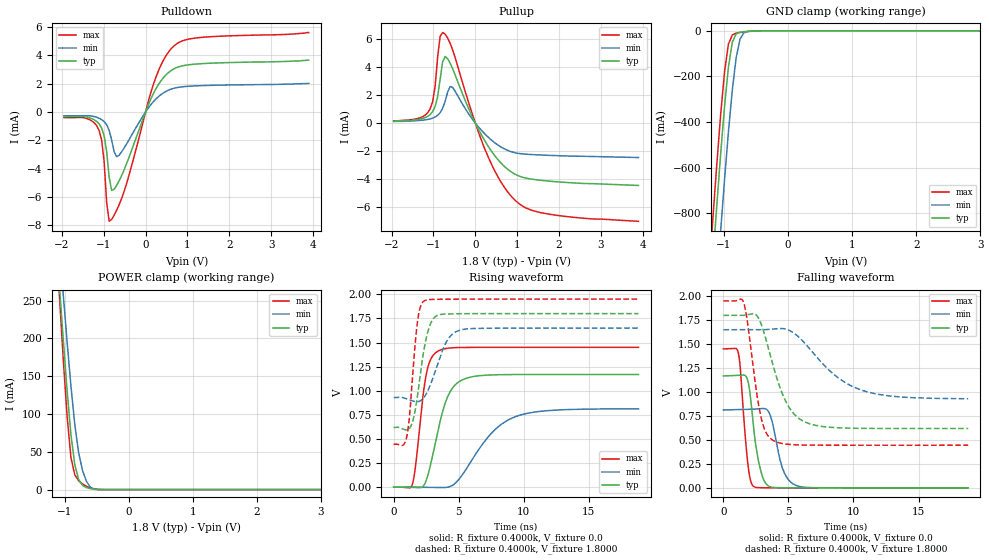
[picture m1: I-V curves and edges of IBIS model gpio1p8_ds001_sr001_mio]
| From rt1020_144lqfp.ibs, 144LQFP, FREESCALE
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[Model] gpio1p8_ds001_sr001_mio
|   Model gpio1p8_ds001_sr001_mio
| This model was characterised for following simulation conditions:
| External (pad) voltage:
|   - Typ: 1.8V,   - Min: 1.65V,   - Max: 1.95V
| Library cells for typ/min/max conditions are connected as defined below:
|  pad - External Pad
|  ipp_do - Core Input
|  ipp_obe - Output Buffer Enable
|  esd_boost - ovdd
|  ipp_dse0 - vddi
|  ipp_dse1 - vssi
|  ipp_dse2 - vssi
|  ipp_fsel0 - vddi
|  ipp_fsel1 - vssi
|  ipp_ina - ipp_ina
|  ipp_ind - ipp_ind
|  ipp_pwr_stable - vddi
|  ipp_sre - vssi
|  ovdd - ovdd
|  ovss - ovss
|  vddi - vddi
|  vssi - vssi
| All other pins connected to ground
Model_type I/O
Polarity   Non-Inverting
Enable   Active-High
Vinl =   0.5400V
Vinh =   1.2600V
Vmeas =  0.9000V
Cref =   0.0F
Rref =   0.4000k
Vref =   0.9000V
C_comp   1.2573pF   1.2208pF   1.3054pF
|C_comp_pullup   0.6439pF   0.6609pF   0.6284pF
|C_comp_pulldown   0.5473pF   0.5786pF   0.5258pF
[Model Spec]
| variable   typ   min   max
Vinh   1.2600V   1.1550V   1.3650V
Vinl   0.5400V   0.4950V   0.5850V
S_overshoot_high   1.8000V   1.6500V   1.9500V
S_overshoot_low   0.0V   0.0V   0.0V
Vmeas   0.9000V   0.8250V   0.9750V
Vref   0.9000V   0.8250V   0.9750V
Cref   0.0F   0.0F   0.0F
Rref   0.4000k   0.4000k   0.4000k
[Temperature Range]   25.0000   0.1050k   -20.0000
[Voltage Range]   1.8000V   1.6500V   1.9500V
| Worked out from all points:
|   slope of the pulldown table from 0 to 0.27 V, typ, clamps not added: 153 ohm
|   slope of the pullup table from 0 to 0.27 V, typ, clamps not added: 182 ohm
|   GND clamp passes 1 mA (typ) near -0.55 V on its own axis
|   POWER clamp passes 1 mA (typ) near -0.58 V on its own axis
|   rising waveform, R_fixture 0.4000k, V_fixture 0.0: 20-80 % time 1.3ns typ, 2.8ns min, 747ps max; typ from 0 V to 1.17 V
|   rising waveform, R_fixture 0.4000k, V_fixture 1.8000: 20-80 % time 809ps typ, 1.19ns min, 547ps max; typ from 0.619 V to 1.8 V
|   falling waveform, R_fixture 0.4000k, V_fixture 0.0: 20-80 % time 681ps typ, 847ps min, 496ps max; typ from 1.17 V to 0 V
|   falling waveform, R_fixture 0.4000k, V_fixture 1.8000: 20-80 % time 1.74ns typ, 3.41ns min, 947ps max; typ from 1.8 V to 0.619 V
[Pulldown]
|Voltage   I(typ)   I(min)   I(max)
-1.95V    -342uA     -265uA     -391uA
-1.41V    -350uA     -258uA     -451uA
-1.11V    -834.5uA   -436uA     -1.299mA
-990mV    -1.66mA    -669.8uA   -3.467mA
-930mV    -2.764mA   -895.4uA   -6.362mA
-870mV    -4.603mA   -1.287mA   -7.724mA
-810mV    -5.539mA   -1.972mA   -7.596mA
-750mV    -5.458mA   -2.817mA   -7.285mA
-630mV    -4.849mA   -3.046mA   -6.544mA
210mV     1.438mA    808.6uA    2.151mA
690mV     3.074mA    1.691mA    4.705mA
3.9V      3.67mA     2.03mA     5.62mA
[Pullup]
|Voltage   I(typ)   I(min)   I(max)
-1.95V    130uA      100uA      140uA
-1.08V    597uA      286uA      991uA
-960mV    1.17mA     422uA      2.604mA
-900mV    1.859mA    544uA      4.683mA
-840mV    3.095mA    733.5uA    6.184mA
-780mV    4.362mA    1.044mA    6.458mA
-720mV    4.75mA     1.549mA    6.347mA
-540mV    3.868mA    2.538mA    5.213mA
240mV     -1.338mA   -819.3uA   -1.942mA
960mV     -3.677mA   -2.134mA   -5.547mA
1.74V     -4.15mA    -2.312mA   -6.505mA
3.9V      -4.465mA   -2.469mA   -7.027mA
[GND_clamp]
|Voltage   I(typ)   I(min)   I(max)
-1.95V    -4.191A    -4.477A    -4.042A
-1.23V    -1.234A    -1.577A    -1.052A
-1.17V    -993.2mA   -1.338A    -811.1mA
-1.11V    -758.1mA   -1.102A    -578.5mA
-1.05V    -533.7mA   -870.8mA   -361.6mA
-990mV    -328mA     -648.8mA   -176.9mA
-930mV    -157.5mA   -441.8mA   -57.56mA
-870mV    -50.13mA   -259.5mA   -18.17mA
-810mV    -13.28mA   -118mA     -10.41mA
-750mV    -5.921mA   -36.52mA   -7.502mA
-630mV    -2.275mA   -2.653mA   -3.283mA
3.9V      0A         0A         0A
[POWER_clamp]
|Voltage   I(typ)   I(min)   I(max)
-1.95V    1.356A     1.328A     1.514A
-1.08V    270.6mA    322.7mA    256.8mA
-1.02V    199mA      258.1mA    173mA
-960mV    131.2mA    195.7mA    97.36mA
-900mV    72.67mA    137.2mA    42.48mA
-840mV    32.99mA    86.34mA    19.5mA
-780mV    13.32mA    48.87mA    11.87mA
-720mV    5.671mA    25.66mA    7.515mA
-660mV    2.793mA    11.19mA    4.477mA
-600mV    1.289mA    3.449mA    2.334mA
-480mV    122.1uA    182.3uA    260.9uA
3.9V      0A         0A         0A
[Ramp]
| variable   typ   min   max
dV/dt_r  0.7010/1.3021n   0.4874/2.8016n   0.8700/0.7474n
dV/dt_f  0.7085/1.7382n   0.4319/3.4124n   0.9031/0.9472n
R_load = 0.4000k
[Rising Waveform]
R_fixture= 0.4000k
V_fixture= 0.0
V_fixture_min= 0.0
V_fixture_max= 0.0
|time   V(typ)   V(min)   V(max)
0s        2.139nV    20.29nV    4.327nV
1.431ns   -2.849mV   235.8uV    26.28mV
1.668ns   -4.299mV   55.34uV    203.6mV
2.507ns   71.79mV    -1.75mV    1.171V
3.411ns   589.2mV    -3.726mV   1.411V
4.292ns   978.8mV    4.565mV    1.443V
5.696ns   1.134V     212.7mV    1.45V
7.842ns   1.165V     603.4mV    1.45V
9.647ns   1.168V     744.4mV    1.45V
18.82ns   1.168V     812.3mV    1.45V
[Rising Waveform]
R_fixture= 0.4000k
V_fixture= 1.8000
V_fixture_min= 1.6500
V_fixture_max= 1.9500
|time   V(typ)   V(min)   V(max)
0s        619.2mV    928.9mV    444.9mV
999.6ps   593.5mV    916.5mV    519.7mV
1.203ns   607.8mV    906.7mV    717.4mV
1.464ns   682.9mV    894.5mV    1.169V
1.814ns   932.2mV    886.5mV    1.699V
2.367ns   1.456V     937.9mV    1.933V
3.126ns   1.759V     1.173V     1.948V
4.136ns   1.796V     1.526V     1.95V
5.143ns   1.799V     1.63V      1.95V
18.82ns   1.8V       1.65V      1.95V
[Falling Waveform]
R_fixture= 0.4000k
V_fixture= 0.0
V_fixture_min= 0.0
V_fixture_max= 0.0
|time   V(typ)   V(min)   V(max)
0s        1.168V     812.6mV    1.45V
1.149ns   1.174V     817.2mV    1.408V
1.91ns    1.101V     819.3mV    216.7mV
2.387ns   550.4mV    821.6mV    9.603mV
2.835ns   197mV      826.4mV    1.793mV
3.311ns   37.03mV    818.8mV    931.6uV
3.673ns   8.04mV     729mV      571.2uV
4.62ns    1.159mV    176.6mV    153.7uV
5.651ns   454uV      21.72mV    34.26uV
18.82ns   16.57nV    2.538uV    17.6nV
[Falling Waveform]
R_fixture= 0.4000k
V_fixture= 1.8000
V_fixture_min= 1.6500
V_fixture_max= 1.9500
|time   V(typ)   V(min)   V(max)
0s        1.8V       1.65V      1.95V
1.549ns   1.8V       1.65V      1.938V
1.845ns   1.807V     1.65V      1.733V
2.442ns   1.813V     1.65V      1.102V
2.897ns   1.711V     1.65V      734.2mV
3.83ns    1.272V     1.658V     494.4mV
5.095ns   829.9mV    1.641V     453mV
6.746ns   663.6mV    1.433V     445.6mV
10.66ns   620.8mV    1.018V     444.9mV
18.82ns   619.2mV    930.1mV    444.9mV
